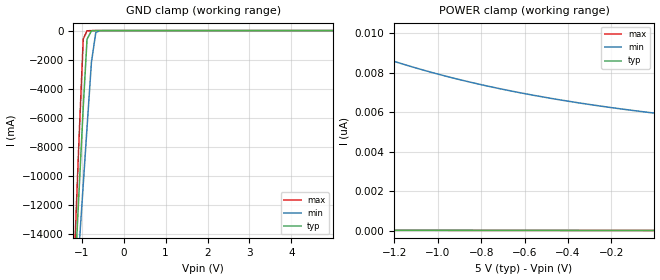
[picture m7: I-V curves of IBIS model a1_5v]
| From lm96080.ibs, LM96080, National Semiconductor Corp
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[Model] a1_5v
Model_type Input
Vinh = 2.0V
Vinl = 0.8V
C_comp   1.18pF   1.09pF   1.34pF
[Voltage Range]   5.0V   4.5V   5.5V
[Temperature Range]   25.0   125.0   -40.0
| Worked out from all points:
|   GND clamp passes 1 mA (typ) near -0.64 V on its own axis
[GND Clamp]
-5V       -239.1A    -186.2A    -298.3A
-1.175V   -17.49A    -19.83A    -15.57A
-1.07V    -11.36A    -15.21A    -7.772A
-965mV    -5.275A    -10.61A    -582.4mA
-875mV    -601.5mA   -6.701A    -16.45mA
-770mV    -16.47mA   -2.184A    -1.94mA
-665mV    -1.247mA   -121.4mA   -149uA
-560mV    -94.18uA   -7.217mA   -5.387uA
-470mV    -7.817uA   -757.7uA   -192.7nA
4.99V     33.83pA    0A         29.94pA
[POWER Clamp]
-5V       181.4pA    85.38nA    63.08pA
-3.575V   95.95pA    33.85nA    54.48pA
-1.61V    49.77pA    10.28nA    42.66pA
-1.565V   49.19pA    10.06nA    42.39pA
-1.415V   47.31pA    9.385nA    41.49pA
-1.205V   44.88pA    8.58nA     40.23pA
-1.055V   43.26pA    8.089nA    39.33pA
-860mV    41.3pA     7.54nA     38.16pA
-650mV    39.33pA    7.043nA    36.9pA
-455mV    37.61pA    6.655nA    35.73pA
-245mV    35.85pA    6.299nA    34.47pA
-5mV      33.94pA    5.956nA    33.03pA
